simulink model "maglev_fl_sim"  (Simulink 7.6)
settings: Solver=ode45  StartTime=0.0  StopTime=5  RelTol=1e-3
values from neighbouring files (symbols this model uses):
  C = C * 1e-5    [maglev_init.m]
  g = 9.80665    [maglev_init.m]
  L1 = L1/10    [maglev_init.m]
  m = m/100    [maglev_init.m]
  R = input('Inserire le prime due cifre (esclusi zeri) del proprio numero di matricola:\n\n')    [maglev_init.m]
  x1_0 = 0.1    [maglev_init.m]
  x1_d = 0.05    [maglev_init.m]
  x2_0 = 0    [maglev_init.m]
  x3_0 = 0.2    [maglev_init.m]
undefined symbols (not defined in the file or in its folder): Ksmc, lambda, mpert
libraries: simulink x1

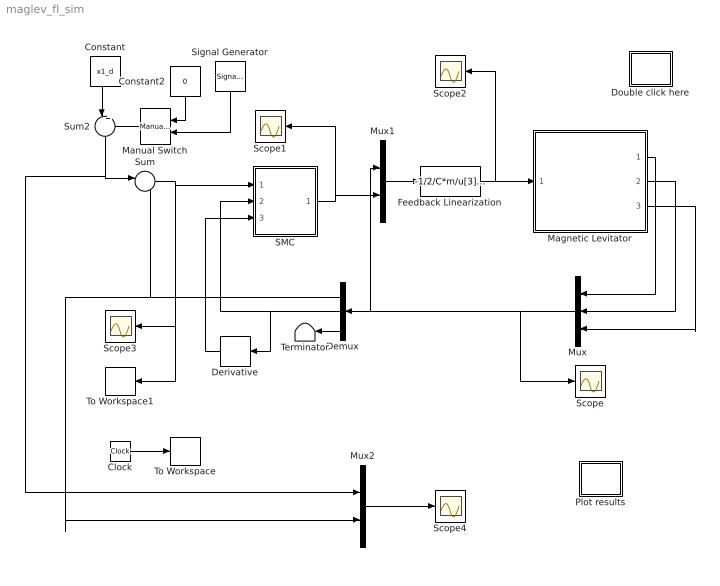
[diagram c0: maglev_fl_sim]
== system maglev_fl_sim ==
  Clock : Clock
  Constant : Constant  Value=x1_d
  Constant2 : Constant  Value=0
  Demux : Demux  Outputs=3
  Derivative : Derivative
  Double click here : Subsystem
  Feedback Linearization : Fcn  Expr=-1/2/C*m/u[3]*u[1]^2*L1*u[4]+u[3]*R-2*C*u[3]/u[1]^2*u[2]+u[3]/u[1]*L1*u[2]
  Magnetic Levitator : Subsystem  mask{m=m+mpert, R=R, L1=L1, C=C, g=g}
      mask prompts: m "ball's mass (m)"; R "Electromagnet's resistance (R)"; L1 "Electromagnet's inductance (L1)"; C "Magnetic force constant (C)"; g "Gravitational acceleration (g)"
  Manual Switch : simulink/Signal Routing/Manual Switch  SystemSampleTime=-1  sw=0  action=0  varsize=off
  Mux : Mux  Inputs=3
  Mux1 : Mux  Inputs=2
  Mux2 : Mux  Inputs=2
  Plot results : Subsystem
  SMC : Subsystem
  Scope{,1..4} (5 alike) : Scope
  Signal Generator : SignalGenerator  WaveForm=square  Amplitude=x1_d*0.1  Frequency=0.5
  Sum : Sum  Inputs=|-+
  Sum2 : Sum  Inputs=|++
  Terminator : Terminator
  To Workspace : ToWorkspace  VariableName=tfl  SampleTime=-1  SaveFormat=Array
  To Workspace1 : ToWorkspace  VariableName=efl  SampleTime=-1  SaveFormat=Array
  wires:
  Magnetic Levitator/1(x1) -> Mux/1
  Magnetic Levitator/2(x2) -> Mux/2
  Magnetic Levitator/3(x3) -> Mux/3
  Mux/1 -> Scope/1, Mux1/1, Demux/1
  Feedback Linearization/1 -> Magnetic Levitator/1(u), Scope2/1
  Constant/1 -> Sum2/1
  Constant2/1 -> Manual Switch/1
  Signal Generator/1 -> Manual Switch/2
  Manual Switch/1 -> Sum2/2
  Mux1/1 -> Feedback Linearization/1
  Sum2/1 -> Sum/1, Mux2/1
  Sum/1 -> Scope3/1, To Workspace1/1, SMC/1(y)
  Derivative/1 -> SMC/3(yddot)
  SMC/1(Out) -> Mux1/2, Scope1/1
  Demux/3 -> Terminator/1
  Demux/1 -> Sum/2, Mux2/2
  Demux/2 -> Derivative/1, SMC/2(ydot)
  Clock/1 -> To Workspace/1
  Mux2/1 -> Scope4/1

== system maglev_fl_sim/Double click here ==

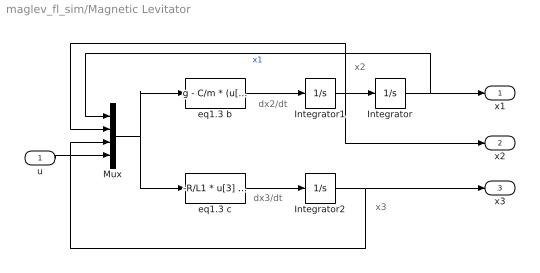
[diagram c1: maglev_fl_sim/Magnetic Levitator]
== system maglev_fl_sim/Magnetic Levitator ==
  note: x2
  note: x3
  note: dx2/dt
  note: dx3/dt
  u : Inport
  Integrator : Integrator  InitialCondition=x1_0
  Integrator1 : Integrator  InitialCondition=x2_0
  Integrator2 : Integrator  InitialCondition=x3_0
  Mux : Mux
  eq1.3 b : Fcn  Expr=g - C/m * (u[3] / u[1])^2
  eq1.3 c : Fcn  Expr=-R/L1 * u[3] + (2*C)/L1 * ( u[2] * u[3] / u[1]^2 ) + 1/L1 * u[4]
  x1 : Outport
  x2 : Outport  Port=2
  x3 : Outport  Port=3
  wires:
  eq1.3 b/1 -> Integrator1/1
  Integrator1/1 -> Integrator/1, Mux/2, x2/1
  eq1.3 c/1 -> Integrator2/1
  Mux/1 -> eq1.3 b/1, eq1.3 c/1
  Integrator/1 -> Mux/1, x1/1  "x1"
  Integrator2/1 -> Mux/3, x3/1
  u/1 -> Mux/4

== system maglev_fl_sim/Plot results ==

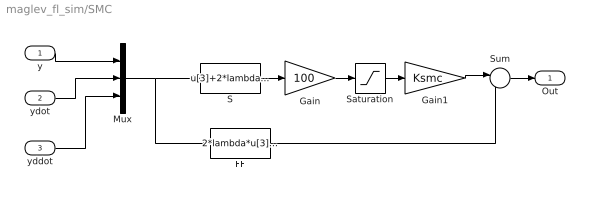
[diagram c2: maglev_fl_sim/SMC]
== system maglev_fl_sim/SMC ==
  y : Inport
  ydot : Inport  Port=2
  yddot : Inport  Port=3
  FF : Fcn  Expr=2*lambda*u[3]+lambda^2*u[2]
  Gain : Gain  Gain=100
  Gain1 : Gain  Gain=Ksmc
  Mux : Mux  Inputs=3
  S : Fcn  Expr=u[3]+2*lambda*u[2]+lambda^2*u[1]
  Saturation : Saturate  UpperLimit=1  LowerLimit=-1
  Sum : Sum  Inputs=|--
  Out : Outport
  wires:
  S/1 -> Gain/1
  Gain/1 -> Saturation/1
  Saturation/1 -> Gain1/1
  Gain1/1 -> Sum/1
  FF/1 -> Sum/2
  Sum/1 -> Out/1
  y/1 -> Mux/1
  ydot/1 -> Mux/2
  yddot/1 -> Mux/3
  Mux/1 -> S/1, FF/1
